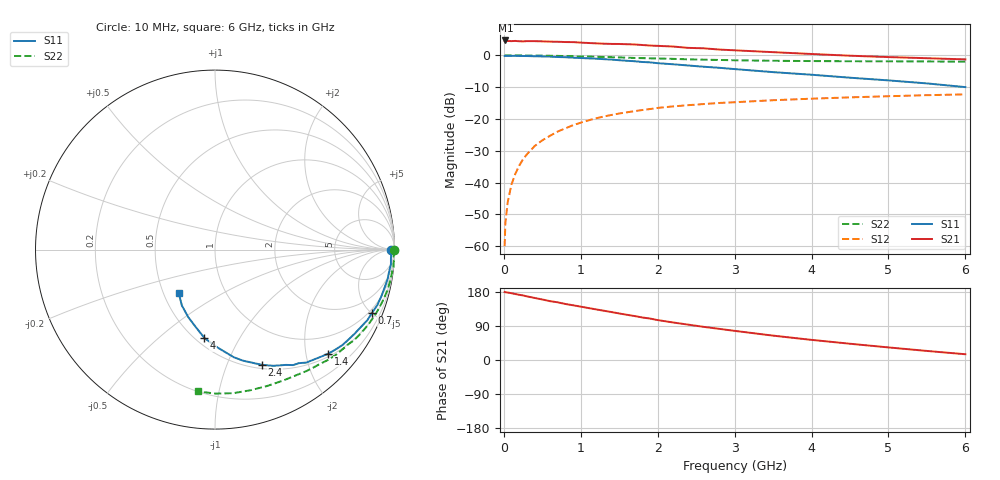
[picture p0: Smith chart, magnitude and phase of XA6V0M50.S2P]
! SIEMENS Discrete & RF Semiconductors
! BFY180
! Si NPN RF Bipolar Junction Transistor in MICRO-X
! VCE = 6 V  IC = 0.5 mA
! Common Emitter S-Parameters:  May  1997
# GHz  S  MA  R  50
!  f  S11  S21  S12  S22
! GHz  MAG  ANG  MAG  ANG  MAG  ANG  MAG  ANG
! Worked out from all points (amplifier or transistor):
!   36 points, 10 MHz to 6 GHz, reference 50 ohm
!   highest |S21| = 4.7 dB at 20 MHz (marker M1)
!   |S21| within 3 dB of that: start of sweep to 2.918 GHz
!   unconditionally stable (mu >= 1): 5.917 GHz to end of sweep
!   at 250 MHz: K = 0.05, MSG = 18.5 dB, |S12| = -32.6 dB
!   at 1.4 GHz: K = 0.38, MSG = 11.2 dB, |S12| = -18.7 dB
!   at 6 GHz: K = 1.00, MAG = 5.1 dB, |S12| = -12.3 dB
!   S11 on the Smith chart (normalised r, x): 10 MHz: 89, -14; 700 MHz: 0.79, -5.00; 1.4 GHz: 0.56, -2.46; 2.4 GHz: 0.54, -1.34; 4 GHz: 0.55, -0.72; 6 GHz: 0.60, -0.33
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0.01  0.9783 -0.2  1.671 179.6  0.001 86.4  0.9993 -0.2
0.02  0.9813 -0.7  1.716 178.8  0.0023 90.0  0.9999 -0.4
0.05  0.9814 -1.4  1.683 178.0  0.0049 82.7  0.9983 -1.0
0.1  0.9817 -3.1  1.676 176.2  0.0094 88.7  0.9957 -2.3
0.2  0.9797 -6.2  1.667 172.1  0.0184 85.7  0.9966 -4.5
0.25  0.9768 -8.1  1.658 170.3  0.0234 84.3  0.9989 -5.6
0.4  0.9682 -12.7  1.673 163.8  0.0375 80.1  0.9934 -8.9
0.6  0.9555 -19.0  1.645 155.3  0.0544 75.1  0.9863 -13.3
0.7  0.9426 -22.1  1.637 152.2  0.0634 72.3  0.9815 -15.4
0.9  0.9203 -27.9  1.616 144.4  0.0799 67.7  0.9697 -19.8
1.1  0.8976 -33.8  1.565 137.1  0.0951 63.4  0.9571 -23.9
1.4  0.8575 -42.5  1.513 126.5  0.1157 56.4  0.9363 -30.0
1.7  0.809 -51.1  1.484 116.0  0.1328 50.7  0.9102 -35.5
2.2  0.7248 -63.3  1.377 99.0  0.1577 41.8  0.8814 -44.1
2.4  0.6928 -67.9  1.312 93.2  0.1648 38.8  0.8656 -47.2
2.6  0.6626 -71.9  1.291 87.4  0.1717 36.0  0.856 -50.1
3  0.6088 -80.1  1.201 76.9  0.1834 30.6  0.8374 -55.8
3.5  0.5451 -88.6  1.123 64.3  0.1971 25.1  0.8226 -62.4
4  0.4962 -96.8  1.051 53.1  0.2085 19.7  0.8136 -69.1
4.5  0.4455 -103.8  0.988 42.9  0.2187 15.0  0.8082 -75.8
5.5  0.3623 -120.6  0.902 23.9  0.2367 5.7  0.8024 -89.7
6  0.3168 -129.5  0.865 15.2  0.2437 0.9  0.7959 -96.7
